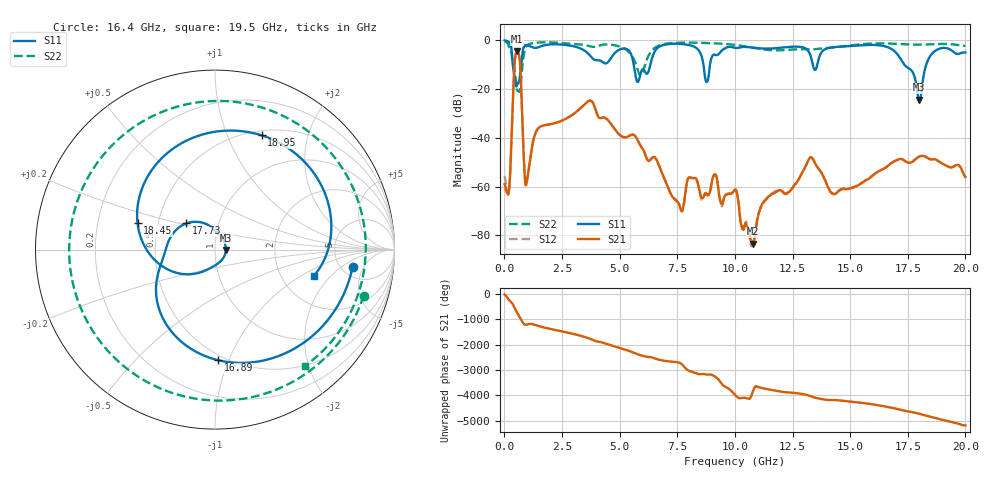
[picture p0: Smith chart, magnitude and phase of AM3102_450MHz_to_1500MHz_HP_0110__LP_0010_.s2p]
!Agilent Technologies,E8364B,MY43040894,A.07.50.67
!Agilent E8364B: A.07.50.67
!Date: Thursday, January 11, 2018 05:45:20
!Correction: S11(Full 2 Port(1,2))
!S21(Full 2 Port(1,2))
!S12(Full 2 Port(1,2))
!S22(Full 2 Port(1,2))
!S2P File: Measurements: S11, S21, S12, S22:
# Hz S  dB  R 50
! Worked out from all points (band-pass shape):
!   1601 points, 10 MHz to 20 GHz, reference 50 ohm
!   highest |S21| = -4.58 dB at 547.2 MHz (marker M1); lowest = -83.5 dB at 10.77 GHz (marker M2)
!   |S21| within 3 dB of the highest: 463.3 MHz to 660.8 MHz (197.5 MHz wide, 35.1 % of centre)
!   lowest |S11| = -24.3 dB at 18 GHz (marker M3), VSWR 1.13, Z = 56.5 - j0.312 ohm
!   |S11| at or under -10 dB: 363.1 MHz to 731.6 MHz (368.6 MHz wide, 67.3 % of centre); 5.61 GHz to 6.332 GHz (722.6 MHz wide, 12.1 % of centre); 17.35 GHz to 18.3 GHz (949 MHz wide, 5.32 % of centre)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
!   |S22| runs from -21.2 to -0.4 dB; largest |S21 - S12| = 0.0013
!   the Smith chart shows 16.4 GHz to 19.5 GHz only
!   S11 on the Smith chart (normalised r, x): 16.4 GHz: 6.28, -3.05; 16.89 GHz: 0.46, -0.92; 17.73 GHz: 0.70, +0.21; 18.45 GHz: 0.38, +0.14; 18.95 GHz: 0.55, +1.34; 19.5 GHz: 3.03, -1.31
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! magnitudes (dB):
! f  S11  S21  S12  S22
! 10 MHz  -0.1  -59.1  -55.7  -0.4
! 209.9 MHz  -0.8  -60.9  -60.6  -2.9
! 547.2 MHz  -18.1  -4.6  -4.6  -20.4
! 959.5 MHz  -2.0  -58.7  -59.1  -2.3
! 1.459 GHz  -2.9  -36.2  -36.2  -0.9
! 3.346 GHz  -3.5  -27.5  -27.5  -1.7
! 6.682 GHz  -2.8  -50.8  -50.7  -2.3
! 7.681 GHz  -1.5  -70.0  -70.2  -1.0
! 8.781 GHz  -17.1  -63.1  -63.3  -1.1
! 10.01 GHz  -3.1  -61.3  -61.2  -1.9
! 10.77 GHz  -3.0  -83.5  -83.6  -3.0
! 13.34 GHz  -8.4  -48.2  -48.2  -3.8
! 14.27 GHz  -2.8  -63.0  -63.1  -2.9
! 16.4 GHz  -2.2  -52.9  -53.0  -1.2
! 16.68 GHz  -3.0  -51.2  -51.2  -1.3
! 16.89 GHz  -4.2  -49.8  -49.9  -1.4
! 17.73 GHz  -13.3  -49.7  -49.6  -1.8
! 18 GHz  -24.3  -47.7  -47.7  -1.8
! 18.45 GHz  -6.8  -48.8  -48.7  -1.7
! 18.95 GHz  -3.3  -50.4  -50.3  -1.5
! 19.5 GHz  -4.9  -51.8  -51.8  -1.7
! 20 GHz  -5.0  -56.1  -56.4  -2.3
